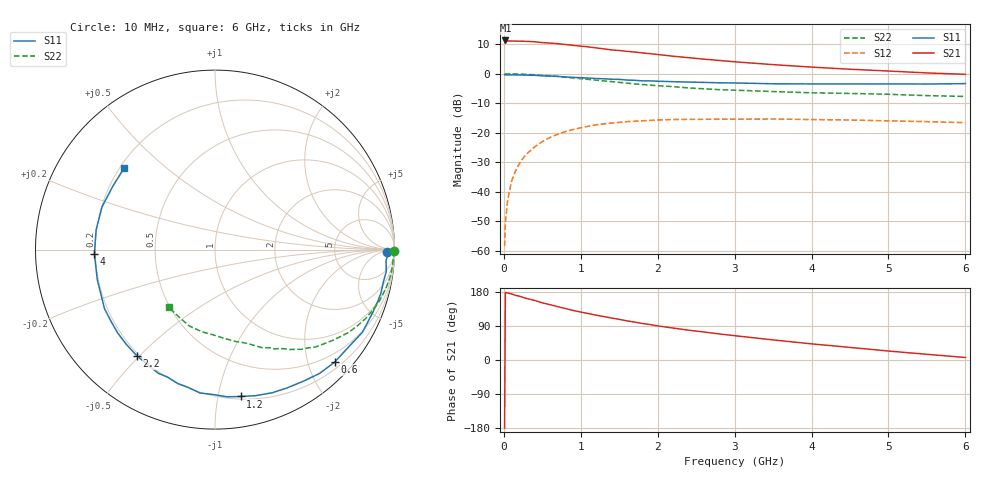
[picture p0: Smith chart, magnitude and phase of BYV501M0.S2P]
! SIEMENS Small Signal Semiconductors
! BFY420
! Si NPN RF SIEGET Grounded Emitter Transistor in MICRO-X
! VCE = 0.5 V  IC = 1 mA
! Common Emitter S-Parameters:  October  1996
# GHz  S  MA  R  50
!  f  S11  S21  S12  S22
! GHz  MAG  ANG  MAG  ANG  MAG  ANG  MAG  ANG
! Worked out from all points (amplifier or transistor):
!   36 points, 10 MHz to 6 GHz, reference 50 ohm
!   highest |S21| = 11.3 dB at 20 MHz (marker M1)
!   |S21| within 3 dB of that: start of sweep to 1.343 GHz
!   unconditionally stable (mu >= 1): 4.519 GHz to end of sweep
!   at 250 MHz: K = 0.05, MSG = 19.8 dB, |S12| = -28.6 dB
!   at 1.4 GHz: K = 0.26, MSG = 12.4 dB, |S12| = -16.7 dB
!   at 6 GHz: K = 1.34, MAG = 4.7 dB, |S12| = -16.6 dB
!   S11 on the Smith chart (normalised r, x): 10 MHz: 41, -15; 600 MHz: 0.32, -2.49; 1.2 GHz: 0.22, -1.17; 2.2 GHz: 0.19, -0.49; 4 GHz: 0.20, -0.02; 6 GHz: 0.22, +0.37
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0.01  0.958 -0.9  3.627 -179.5  0.0012 87.4  0.9988 -0.5
0.02  0.9621 -1.6  3.666 178.5  0.003 92.7  0.9967 -0.9
0.05  0.9552 -3.8  3.588 176.6  0.0073 88.6  0.9959 -2.2
0.1  0.962 -7.3  3.589 174.5  0.0151 84.5  0.9932 -4.4
0.15  0.9552 -10.9  3.576 170.6  0.0222 81.9  0.9908 -6.5
0.2  0.9558 -14.7  3.567 168.5  0.0297 80.9  0.9879 -8.6
0.3  0.9461 -21.8  3.535 162.1  0.0442 75.8  0.9762 -12.9
0.4  0.9419 -29.2  3.482 157.3  0.0577 71.2  0.9616 -16.9
0.5  0.921 -36.1  3.37 150.8  0.071 66.6  0.9422 -20.9
0.6  0.9151 -43.2  3.309 146.0  0.0833 62.2  0.9224 -24.7
0.8  0.883 -56.2  3.133 135.8  0.1048 53.6  0.8754 -31.8
1.1  0.8445 -74.6  2.853 122.5  0.1292 42.8  0.8012 -41.0
1.2  0.8305 -80.1  2.739 118.3  0.1365 39.4  0.7803 -44.0
1.4  0.8075 -90.6  2.535 110.7  0.146 33.3  0.737 -48.9
1.8  0.7583 -110.2  2.258 96.4  0.1596 23.5  0.6577 -57.0
2.2  0.7345 -126.4  1.984 84.3  0.1676 14.9  0.605 -64.5
2.8  0.7031 -146.0  1.681 68.8  0.1702 5.7  0.5378 -73.9
3.5  0.6771 -165.6  1.428 53.0  0.1712 -2.3  0.4996 -83.4
4  0.6723 -178.1  1.297 42.6  0.1675 -7.1  0.4758 -91.0
4.5  0.6715 170.5  1.193 33.2  0.1645 -11.6  0.4635 -98.9
5.5  0.6701 147.9  1.033 15.0  0.1544 -17.3  0.4264 -117.9
6  0.6809 137.8  0.978 6.6  0.1485 -18.4  0.4123 -128.7
